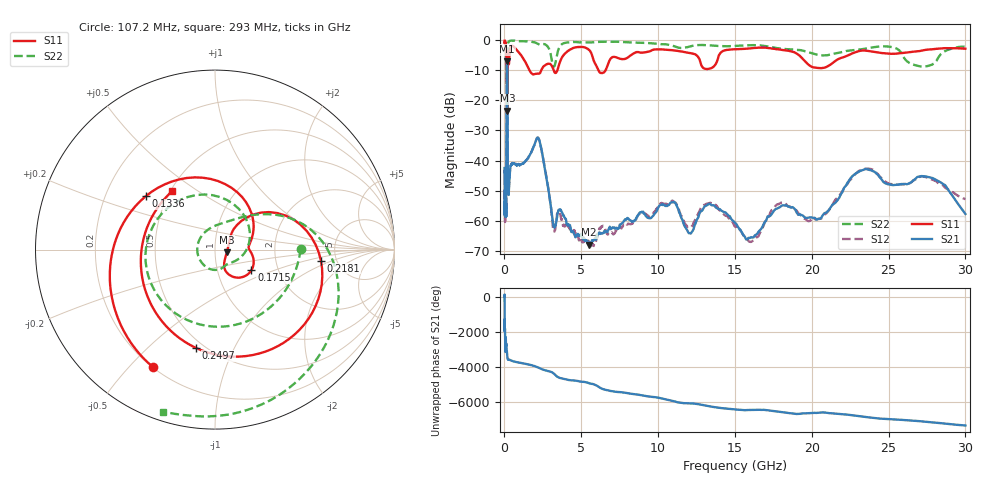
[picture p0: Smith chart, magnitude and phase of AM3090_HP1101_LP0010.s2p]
! Date/Time: Thu, Feb 28, 2019 2:07 PM
! Network Analyzer: Agilent Technologies E8364B Rev: A.07.50.67
! Sweep from 0.010 to 30.000 GHz, 1601 Points, Sweep Type: LOG
! Power Supply: 5.022 V, 0.002 A
# Hz S DB R 50
!freq MagS11 AngS11 MagS21 AngS21 MagS12 AngS12 MagS22 AngS22
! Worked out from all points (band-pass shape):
!   1601 points, 10 MHz to 30 GHz, reference 50 ohm
!   highest |S21| = -7.11 dB at 167.3 MHz (marker M1); lowest = -67.9 dB at 5.501 GHz (marker M2)
!   |S21| within 3 dB of the highest: 148.8 MHz to 189.9 MHz (41.02 MHz wide, 24.2 % of centre)
!   lowest |S11| = -23.4 dB at 193.4 MHz (marker M3), VSWR 1.14, Z = 57 - j1.68 ohm
!   |S11| at or under -10 dB: 1.618 GHz to 2.398 GHz (780.2 MHz wide, 38.8 % of centre); 3.204 GHz to 3.449 GHz (245.2 MHz wide, 7.37 % of centre); 6.108 GHz to 6.585 GHz (476.8 MHz wide, 7.51 % of centre)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
!   |S22| runs from -20.1 to -0.1 dB; largest |S21 - S12| = 0.012
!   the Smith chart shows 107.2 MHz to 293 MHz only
!   S11 on the Smith chart (normalised r, x): 107.2 MHz: 0.20, -0.58; 133.6 MHz: 0.38, +0.30; 171.5 MHz: 1.46, -0.35; 218.1 MHz: 3.77, -0.71; 249.7 MHz: 0.45, -0.72; 293 MHz: 0.51, +0.40
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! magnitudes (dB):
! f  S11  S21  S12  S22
! 10 MHz  -0.3  -42.5  -45.1  -0.5
! 38.04 MHz  -0.4  -58.1  -58.5  -1.2
! 48.61 MHz  -0.5  -49.5  -49.5  -1.3
! 107.2 MHz  -2.6  -57.4  -53.8  -6.4
! 118.5 MHz  -3.7  -53.1  -53.7  -7.3
! 133.6 MHz  -6.2  -27.6  -27.6  -8.8
! 144.7 MHz  -10.4  -13.0  -13.0  -13.3
! 167.3 MHz  -12.9  -7.1  -7.1  -18.9
! 171.5 MHz  -12.7  -7.2  -7.2  -19.4
! 193.4 MHz  -23.4  -12.0  -12.0  -13.9
! 218.1 MHz  -4.5  -45.2  -46.0  -2.5
! 249.7 MHz  -5.1  -50.7  -49.5  -0.8
! 293 MHz  -7.9  -49.9  -48.2  -0.5
! 550.5 MHz  -2.1  -40.8  -41.0  -0.3
! 2.084 GHz  -11.2  -32.9  -32.9  -1.0
! 3.188 GHz  -9.8  -61.3  -63.2  -8.8
! 5.501 GHz  -3.3  -67.9  -67.6  -0.8
! 7.926 GHz  -6.1  -59.4  -61.0  -0.8
! 13.34 GHz  -9.5  -54.4  -54.1  -1.7
! 16.13 GHz  -2.7  -65.5  -66.8  -1.7
! 23.48 GHz  -3.5  -42.9  -42.7  -2.9
! 30 GHz  -2.9  -57.7  -52.8  -2.2
